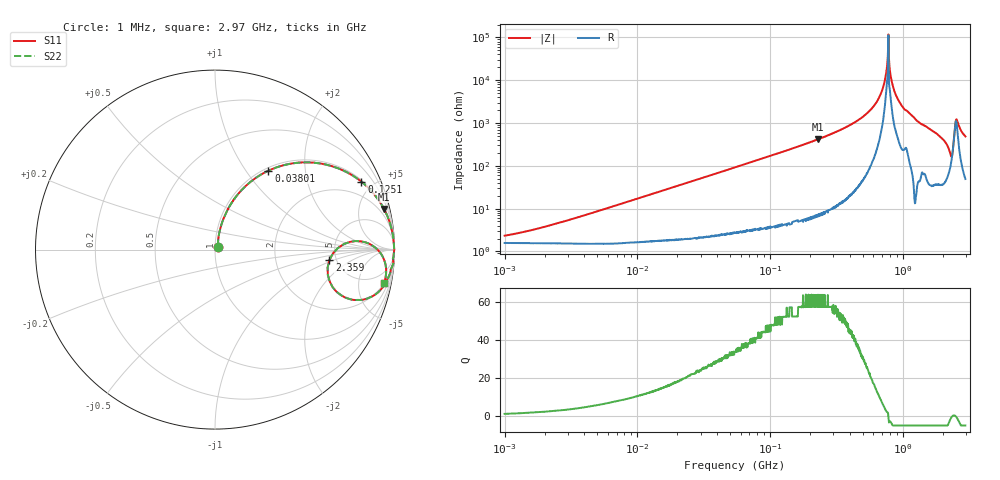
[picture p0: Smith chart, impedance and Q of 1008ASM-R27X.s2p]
!s-Parameter Generated by FASTRON Sdn. Bhd.
!FASTRON P/N : 1008ASM-R27X
!Keysight Technologies: E4991B_MY54100416_A.01.15
!Date: Tue Nov 21 09:05:49 2023
!Version  :Rev00  Wed Nov 22 15:14:05 2023
!Data & Calibration Information:
!Freq  S11  S21  S12  S22
!PortZ  Port1:50+j0  Port2:50+j0
!When reading reference impedance value at option line is always used.
! Remarks : This data is being provided solely for informational purposes.
# Hz S dB R 50
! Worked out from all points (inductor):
!   1599 points, 1 MHz to 2.97 GHz, reference 50 ohm
!   read as one part in series: L = 272 nH near 2.693 MHz
!   highest Q = 63.5 at 229.1 MHz (marker M1), where L = 287 nH
!   self-resonance near 776.9 MHz
!   S11 on the Smith chart (normalised r, x): 1 MHz: 1.03, +0.03; 38.01 MHz: 1.05, +1.28; 125.1 MHz: 1.08, +4.27; 2.359 GHz: 4.37, -0.87; 2.97 GHz: 1.99, -9.70
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1000000  -32.80 46.5  -0.14 -1.0  -0.14 -1.0  -32.80 46.5
3804036  -23.70 73.3  -0.15 -3.7  -0.15 -3.7  -23.70 73.3
1.439846e7  -12.60 72.4  -0.40 -13.5  -0.40 -13.5  -12.60 72.4
3.801167e7  -5.50 55.9  -1.63 -32.1  -1.63 -32.1  -5.50 55.9
5.477226e7  -3.50 46.4  -2.80 -41.9  -2.80 -41.9  -3.50 46.4
1.250659e8  -0.93 24.9  -7.51 -64.0  -7.51 -64.0  -0.93 24.9
2.073156e8  -0.34 15.1  -11.70 -74.0  -11.70 -74.0  -0.34 15.1
2.291374e8  -0.28 13.5  -12.60 -75.6  -12.60 -75.6  -0.28 13.5
4.094372e8  -0.07 6.1  -19.40 -82.6  -19.40 -82.6  -0.07 6.1
5.696638e8  -0.03 2.9  -26.10 -84.4  -26.10 -84.4  -0.03 2.9
6.889699e8  -0.02 1.1  -34.10 -81.7  -34.10 -81.7  -0.02 1.1
7.316083e8  -0.02 0.6  -39.50 -75.8  -39.50 -75.8  -0.02 0.6
7.614901e8  -0.02 0.3  -46.20 -63.1  -46.20 -63.1  -0.02 0.3
7.846996e8  -0.01 -0.1  -54.70 65.2  -54.70 65.2  -0.01 -0.1
8.586597e8  -0.02 -0.9  -35.70 79.6  -35.70 79.6  -0.02 -0.9
1.002744e9  -0.04 -2.4  -27.50 81.8  -27.50 81.8  -0.04 -2.4
1.837163e9  -0.25 -10.3  -14.90 75.8  -14.90 75.8  -0.25 -10.3
2.199798e9  -1.11 -18.3  -9.87 59.2  -9.87 59.2  -1.11 -18.3
2.359433e9  -3.88 -5.3  -8.70 9.2  -8.70 9.2  -3.88 -5.3
2.443543e9  -1.53 2.8  -15.50 -14.1  -15.50 -14.1  -1.53 2.8
2.556106e9  -0.54 -3.0  -22.20 38.4  -22.20 38.4  -0.54 -3.0
2.970126e9  -0.35 -11.3  -14.10 72.9  -14.10 72.9  -0.35 -11.3
